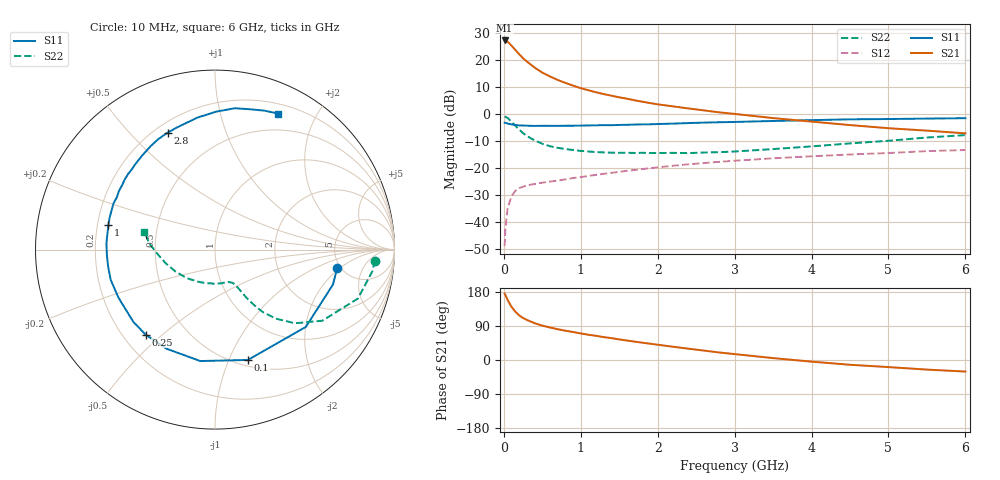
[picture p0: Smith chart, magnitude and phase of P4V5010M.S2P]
! SIEMENS Small Signal Semiconductors
! BFP182
! Si NPN RF Bipolar Junction Transistor in SOT143
! VCE = 0.5 V  IC = 10 mA
! Common Emitter S-Parameters:  March  1996
# GHz  S  MA  R  50
!  f  S11  S21  S12  S22
! GHz  MAG  ANG  MAG  ANG  MAG  ANG  MAG  ANG
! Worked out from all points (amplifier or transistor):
!   36 points, 10 MHz to 6 GHz, reference 50 ohm
!   highest |S21| = 27.2 dB at 10 MHz (marker M1)
!   |S21| within 3 dB of that: start of sweep to 133.3 MHz
!   unconditionally stable (mu >= 1): 555 MHz to end of sweep
!   at 250 MHz: K = 0.53, MSG = 23.7 dB, |S12| = -26.9 dB
!   at 1.4 GHz: K = 1.64, MAG = 9.6 dB, |S12| = -21.8 dB
!   at 6 GHz: K = 1.46, MAG = -0.9 dB, |S12| = -13.3 dB
!   S11 on the Smith chart (normalised r, x): 10 MHz: 4.68, -1.83; 100 MHz: 0.56, -1.18; 250 MHz: 0.29, -0.44; 1 GHz: 0.25, +0.11; 2.8 GHz: 0.25, +0.64; 6 GHz: 0.30, +1.52
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0.01  0.6886 -8.6  22.83 175.5  0.0036 81.7  0.8929 -3.9
0.02  0.6856 -16.5  22.77 171.3  0.0077 82.6  0.8848 -7.9
0.05  0.6645 -40.4  21.58 158.0  0.0182 70.9  0.8417 -18.9
0.1  0.6415 -73.4  18.27 140.3  0.0302 55.2  0.7176 -33.5
0.15  0.6263 -97.5  15.21 127.4  0.0381 47.0  0.6053 -42.7
0.2  0.6147 -116.0  12.68 117.8  0.0427 41.0  0.514 -48.5
0.25  0.6114 -129.2  10.69 110.8  0.0451 37.7  0.4415 -52.4
0.3  0.6076 -138.4  9.285 105.7  0.0479 35.5  0.3911 -54.4
0.4  0.6007 -153.4  7.198 97.1  0.0508 33.6  0.3249 -56.7
0.5  0.605 -163.8  5.811 90.8  0.0537 33.1  0.2811 -57.9
0.6  0.6029 -171.0  4.938 85.7  0.0563 33.8  0.2535 -58.8
0.7  0.6031 -177.3  4.253 81.3  0.0585 34.6  0.2365 -59.6
0.8  0.6059 176.8  3.756 77.3  0.0619 35.0  0.2248 -60.3
1  0.6092 167.0  2.999 70.1  0.0678 36.7  0.2077 -62.7
1.1  0.6136 163.2  2.74 66.6  0.0718 37.0  0.2025 -64.6
1.5  0.6266 148.9  2.03 54.3  0.0851 37.9  0.1919 -71.9
2.2  0.6629 127.7  1.38 35.0  0.1104 35.8  0.1909 -90.6
2.8  0.7028 112.1  1.071 19.8  0.1304 31.7  0.1966 -111.1
3.5  0.7416 97.7  0.839 5.0  0.1514 25.9  0.2243 -135.0
4.5  0.7953 82.0  0.623 -12.6  0.1781 17.6  0.2856 -164.7
5.5  0.8214 70.5  0.492 -25.3  0.2057 9.3  0.3669 174.9
6  0.8353 65.2  0.438 -30.5  0.2154 4.4  0.4066 165.7
